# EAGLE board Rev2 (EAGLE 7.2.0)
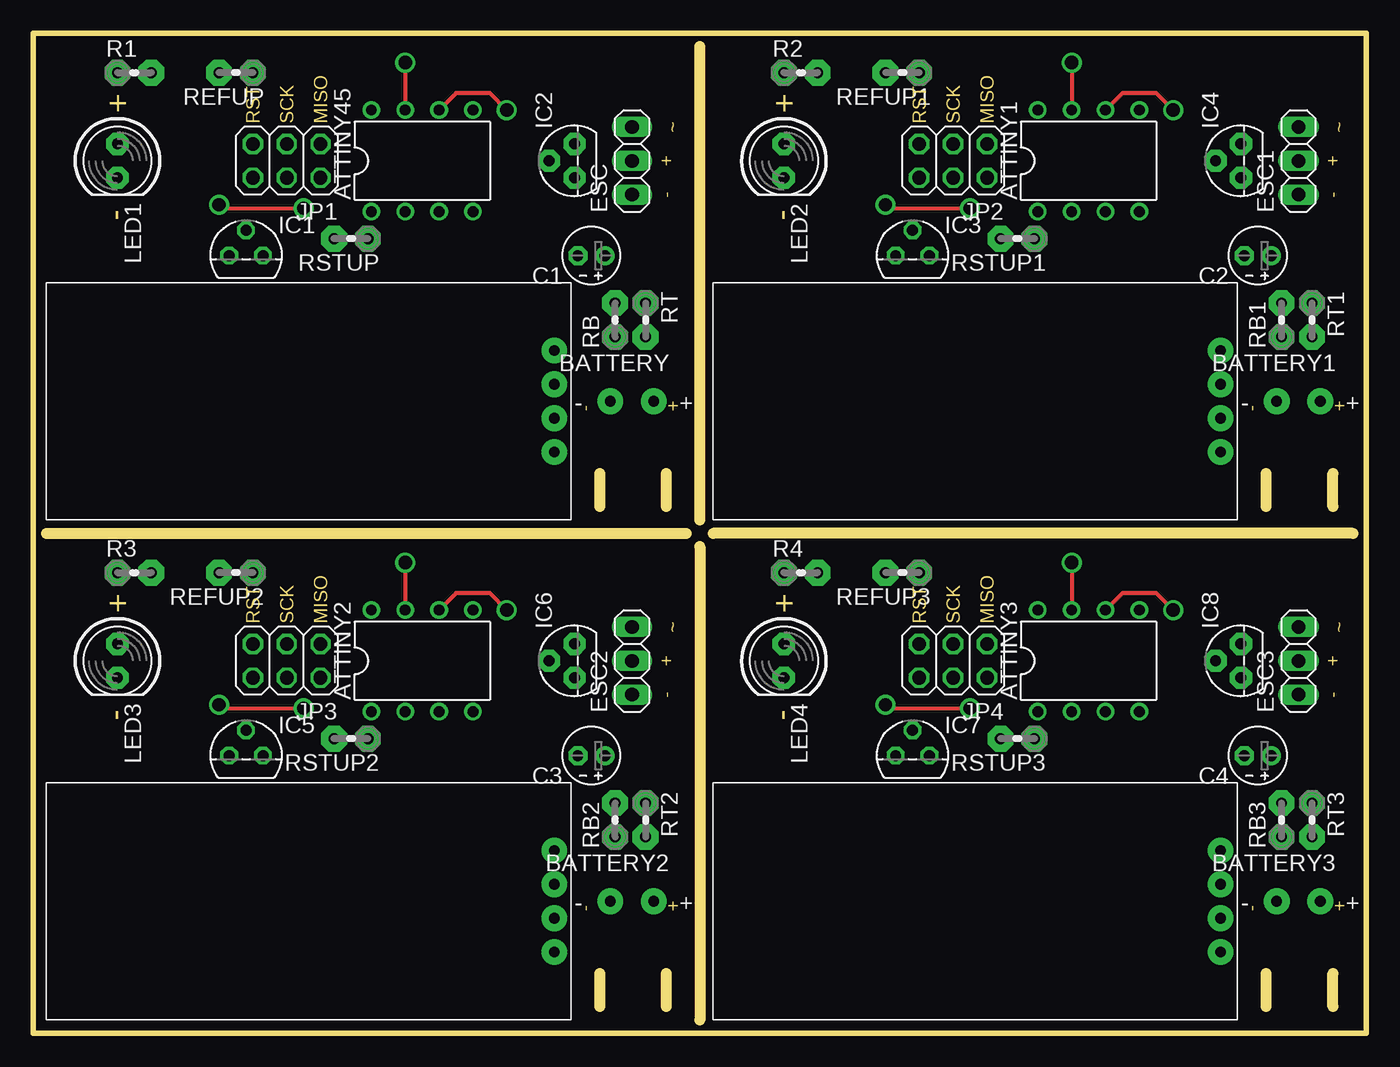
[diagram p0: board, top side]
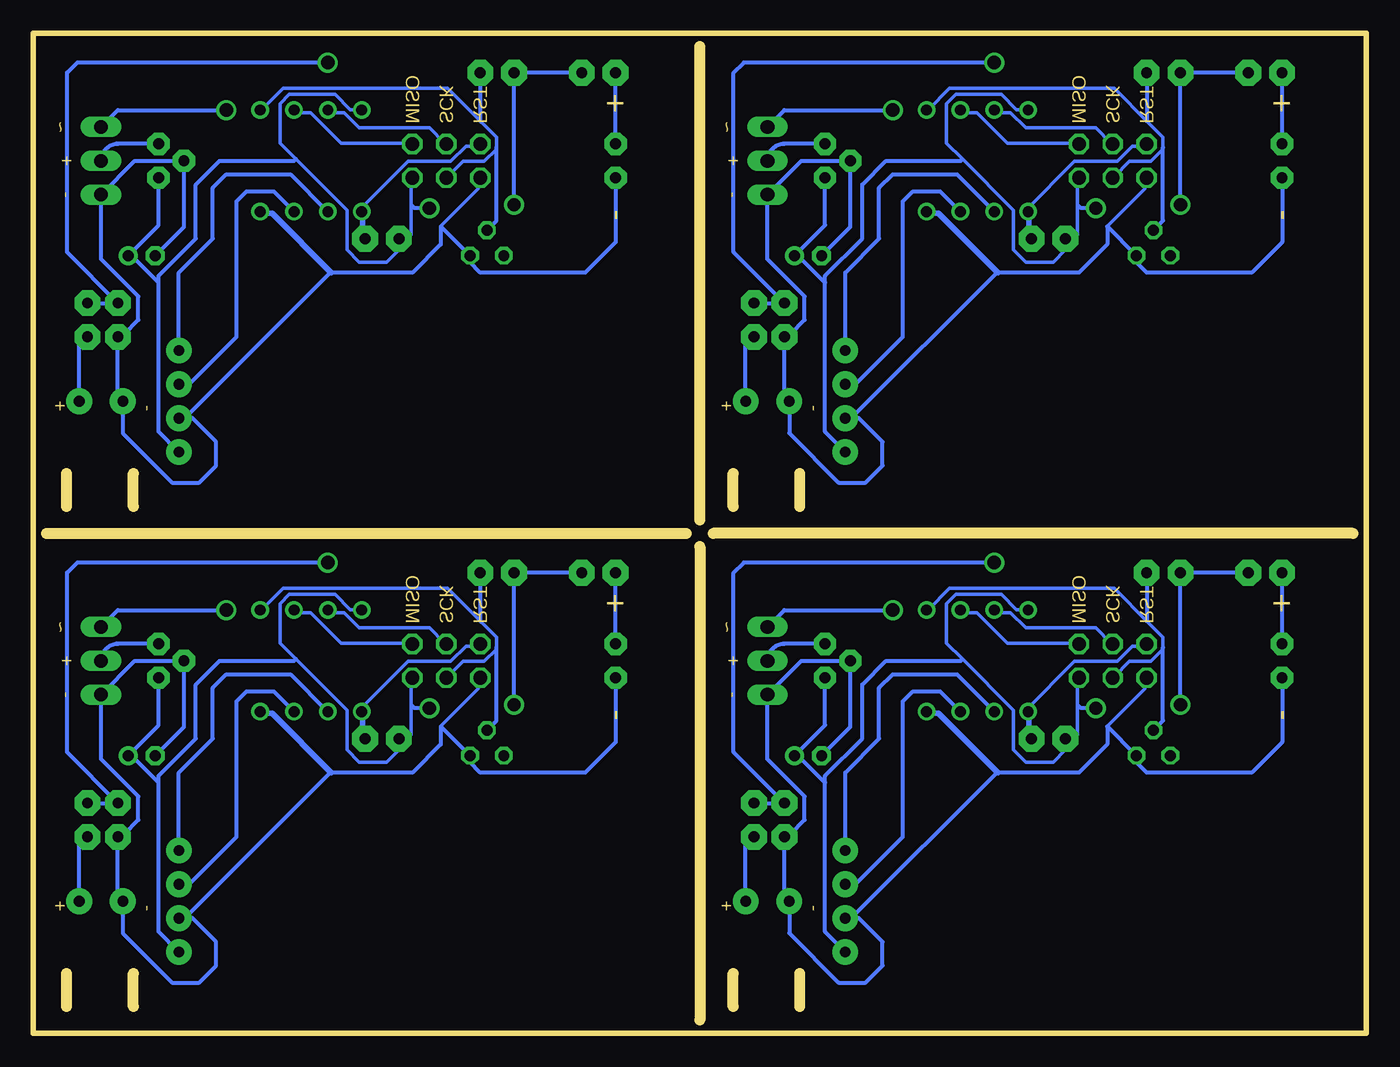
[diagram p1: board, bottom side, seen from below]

Size 100 x 75 mm. Coordinates in mm from the lower left corner, seen from the top.
Outline: 0,75 0,0 100,0 100,75 0,75
Copper layers (1*16): Top 0.035mm / dielectric 1.5mm / Bottom 0.035mm
Design rules "default": minimum track width 10mil, minimum drill 24mil, track to track 8mil, track to pad 8mil, pad to pad 8mil, via to via 8mil, smd to smd 8mil, copper to edge 40mil, drill to drill 8mil, minimum pad ring 10mil, minimum via ring 8mil, stop-mask expansion 4mil, vias tented up to drill 0mil, thermal gap 10mil
Milling: 12 lines

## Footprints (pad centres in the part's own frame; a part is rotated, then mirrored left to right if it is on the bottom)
DIL08 = drill 0.813 pad 1.27: 1 -3.81,-3.81; 2 -1.27,-3.81; 3 1.27,-3.81; 4 3.81,-3.81; 5 3.81,3.81; 6 1.27,3.81; 7 -1.27,3.81; 8 -3.81,3.81
JST-PH-2-THM = drill 0.8 pad 1.93: 1 1.635,0; 2 -1.635,0
E2-4 = drill 0.813 pad 1.422: + -1.016,0 | drill 0.813 pad 1.422 octagon: - 1.016,0
1X03 = drill 1.016 long: 1 -2.54,0; 2 0,0; 3 2.54,0
BT = drill 0.8 pad 1.93: GND -1.27,0; RX 3.81,0; TX 1.27,0; VCC -3.81,0
TO92 = drill 0.813 octagon: 1 -1.27,0; 2 0,1.905; 3 1.27,0
TO92' = drill 0.813 pad 1.676 octagon: 1 -1.27,0; 2 0,1.905; 3 1.27,0
2X03 = drill 1.016 octagon: 1 -2.54,-1.27; 2 -2.54,1.27; 3 0,-1.27; 4 0,1.27; 5 2.54,-1.27; 6 2.54,1.27
LED5MM = drill 0.813 pad 1.676 octagon: A -1.27,0; K 1.27,0
0204V = drill 0.813 pad 1.93 octagon: 1 -1.27,0; 2 1.27,0

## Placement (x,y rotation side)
ATTINY1  ATTINY45DIP8  [DIL08]  79.17,65.44 0 top
ATTINY2  ATTINY45DIP8  [DIL08]  29.17,27.94 0 top
ATTINY3  ATTINY45DIP8  [DIL08]  79.17,27.94 0 top
ATTINY45  ATTINY45DIP8  [DIL08]  29.17,65.44 0 top
BATTERY  [JST-PH-2-THM]  44.92,47.41 180 top
BATTERY1  [JST-PH-2-THM]  94.92,47.41 180 top
BATTERY2  [JST-PH-2-THM]  44.92,9.91 180 top
BATTERY3  [JST-PH-2-THM]  94.92,9.91 180 top
C1  0.1uf  [E2-4]  41.87,58.33 180 top
C2  0.1uf  [E2-4]  91.87,58.33 180 top
C3  0.1uf  [E2-4]  41.87,20.83 180 top
C4  0.1uf  [E2-4]  91.87,20.83 180 top
ESC  [1X03]  44.92,65.44 90 top
ESC1  [1X03]  94.92,65.44 90 top
ESC2  [1X03]  44.92,27.94 90 top
ESC3  [1X03]  94.92,27.94 90 top
HC-01  HC-O6  [BT]  89.08,47.41 90 top
HC-02  HC-O6  [BT]  39.08,9.91 90 top
HC-03  HC-O6  [BT]  89.08,9.91 90 top
HC-06  HC-O6  [BT]  39.08,47.41 90 top
IC1  LM336LP  [TO92]  15.96,58.33 0 top
IC2  78L05Z  [TO92']  40.6,65.44 90 top
IC3  LM336LP  [TO92]  65.96,58.33 0 top
IC4  78L05Z  [TO92']  90.6,65.44 90 top
IC5  LM336LP  [TO92]  15.96,20.83 0 top
IC6  78L05Z  [TO92']  40.6,27.94 90 top
IC7  LM336LP  [TO92]  65.96,20.83 0 top
IC8  78L05Z  [TO92']  90.6,27.94 90 top
JP1  [2X03]  19.01,65.44 180 top
JP2  [2X03]  69.01,65.44 180 top
JP3  [2X03]  19.01,27.94 180 top
JP4  [2X03]  69.01,27.94 180 top
LED1  [LED5MM]  6.31,65.44 270 top
LED2  [LED5MM]  56.31,65.44 270 top
LED3  [LED5MM]  6.31,27.94 270 top
LED4  [LED5MM]  56.31,27.94 270 top
R1  270  [0204V]  7.58,72.04 0 top
R2  270  [0204V]  57.58,72.04 0 top
R3  270  [0204V]  7.58,34.54 0 top
R4  270  [0204V]  57.58,34.54 0 top
RB  20000  [0204V]  43.65,53.5 90 top
RB1  20000  [0204V]  93.65,53.5 90 top
RB2  20000  [0204V]  43.65,16 90 top
RB3  20000  [0204V]  93.65,16 90 top
REFUP  2200  [0204V]  15.2,72.04 180 top
REFUP1  2200  [0204V]  65.2,72.04 180 top
REFUP2  2200  [0204V]  15.2,34.54 180 top
REFUP3  2200  [0204V]  65.2,34.54 180 top
RSTUP  10000  [0204V]  23.84,59.6 180 top
RSTUP1  10000  [0204V]  73.84,59.6 180 top
RSTUP2  10000  [0204V]  23.84,22.1 180 top
RSTUP3  10000  [0204V]  73.84,22.1 180 top
RT  220000  [0204V]  45.94,53.5 270 top
RT1  220000  [0204V]  95.94,53.5 270 top
RT2  220000  [0204V]  45.94,16 270 top
RT3  220000  [0204V]  95.94,16 270 top

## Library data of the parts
ATTINY1-ATTINY3 ATTINY45 HC-01-HC-03 HC-06 IC1 IC3 IC5 IC7 = VLADLIBRARY
BATTERY BATTERY1-BATTERY3 C1-C4 IC2 IC4 IC6 IC8 LED1-LED4 R1-R4 RB RB1-RB3 REFUP REFUP1-REFUP3 RSTUP RSTUP1-RSTUP3 RT RT1-RT3 = adafruit
ESC ESC1-ESC3 JP1-JP4 = pinhead

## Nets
CONTROL: ATTINY45.6 ESC.3 JP1.1
CONTROL1: ATTINY1.6 ESC1.3 JP2.1
CONTROL2: ATTINY2.6 ESC2.3 JP3.1
CONTROL3: ATTINY3.6 ESC3.3 JP4.1
GND: ATTINY45.4 BATTERY.1 C1.- ESC.1 HC-06.GND IC1.3 IC2.2 JP1.6 LED1.K RB.1
GND1: ATTINY1.4 BATTERY1.1 C2.- ESC1.1 HC-01.GND IC3.3 IC4.2 JP2.6 LED2.K RB1.1
GND2: ATTINY2.4 BATTERY2.1 C3.- ESC2.1 HC-02.GND IC5.3 IC6.2 JP3.6 LED3.K RB2.1
GND3: ATTINY3.4 BATTERY3.1 C4.- ESC3.1 HC-03.GND IC7.3 IC8.2 JP4.6 LED4.K RB3.1
N$1: ESC.2 IC2.3
N$2: LED1.A R1.1
N$3: ATTINY45.1 JP1.5 RSTUP.1
N$4: BATTERY.2 RT.2
N$5: ATTINY1.1 JP2.5 RSTUP1.1
N$6: ESC1.2 IC4.3
N$7: BATTERY1.2 RT1.2
N$8: LED2.A R2.1
N$9: ATTINY2.1 JP3.5 RSTUP2.1
N$10: ESC2.2 IC6.3
N$11: BATTERY2.2 RT2.2
N$12: LED3.A R3.1
N$13: ATTINY3.1 JP4.5 RSTUP3.1
N$14: ESC3.2 IC8.3
N$15: BATTERY3.2 RT3.2
N$16: LED4.A R4.1
RX: ATTINY45.3 HC-06.TX
RX1: ATTINY1.3 HC-01.TX
RX2: ATTINY2.3 HC-02.TX
RX3: ATTINY3.3 HC-03.TX
TX: ATTINY45.2 HC-06.RX
TX1: ATTINY1.2 HC-01.RX
TX2: ATTINY2.2 HC-02.RX
TX3: ATTINY3.2 HC-03.RX
VCC: ATTINY45.8 C1.+ HC-06.VCC IC2.1 JP1.2 R1.2 REFUP.2 RSTUP.2
VCC1: ATTINY1.8 C2.+ HC-01.VCC IC4.1 JP2.2 R2.2 REFUP1.2 RSTUP1.2
VCC2: ATTINY2.8 C3.+ HC-02.VCC IC6.1 JP3.2 R3.2 REFUP2.2 RSTUP2.2
VCC3: ATTINY3.8 C4.+ HC-03.VCC IC8.1 JP4.2 R4.2 REFUP3.2 RSTUP3.2
VOLTMETER: ATTINY45.7 JP1.3 RB.2 RT.1
VOLTMETER1: ATTINY1.7 JP2.3 RB1.2 RT1.1
VOLTMETER2: ATTINY2.7 JP3.3 RB2.2 RT2.1
VOLTMETER3: ATTINY3.7 JP4.3 RB3.2 RT3.1
VREF: ATTINY45.5 IC1.2 JP1.4 REFUP.1
VREF1: ATTINY1.5 IC3.2 JP2.4 REFUP1.1
VREF2: ATTINY2.5 IC5.2 JP3.4 REFUP2.1
VREF3: ATTINY3.5 IC7.2 JP4.4 REFUP3.1

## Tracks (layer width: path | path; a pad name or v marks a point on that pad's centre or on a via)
CONTROL  (via drill 1)
  Top 0.305: v35.52,69.25 34.25,70.52 31.71,70.52 ATTINY45.6
  Bottom 0.254: ATTINY45.6 30.34,69.05 29.2,69.05 26.91,66.76 21.65,66.76 JP1.1
  Bottom 0.305: ESC.3 43.65,69.25 v35.52,69.25
CONTROL1  (via drill 1)
  Top 0.305: v85.52,69.25 84.25,70.52 81.71,70.52 ATTINY1.6
  Bottom 0.254: ATTINY1.6 80.34,69.05 79.2,69.05 76.91,66.76 71.65,66.76 JP2.1
  Bottom 0.305: ESC1.3 93.65,69.25 v85.52,69.25
CONTROL2  (via drill 1)
  Top 0.305: v35.52,31.75 34.25,33.02 31.71,33.02 ATTINY2.6
  Bottom 0.254: ATTINY2.6 30.34,31.55 29.2,31.55 26.91,29.26 21.65,29.26 JP3.1
  Bottom 0.305: ESC2.3 43.65,31.75 v35.52,31.75
CONTROL3  (via drill 1)
  Top 0.305: v85.52,31.75 84.25,33.02 81.71,33.02 ATTINY3.6
  Bottom 0.254: ATTINY3.6 80.34,31.55 79.2,31.55 76.91,29.26 71.65,29.26 JP4.1
  Bottom 0.305: ESC3.3 93.65,31.75 v85.52,31.75
GND
  Bottom 0.254: 19.43,60.52 16.62,63.33 16.62,64.02 JP1.6 | 32.85,61.5 ATTINY45.4
  Bottom 0.305: C1.- 38.7,60.49 IC2.2 42.38,65.44 ESC.1 44.92,58.07 42.13,55.28 42.13,53.5 43.14,52.49 43.4,52.49 RB.1 43.65,47.68 BATTERY.1 43.28,45.01 39.59,41.31 37.55,41.31 36.28,42.58 36.28,44.36 38.06,46.14 HC-06.GND 38.65,46.14 27.72,57.06 27.65,57.06 21.55,57.06 19.43,59.18 19.43,60.52 IC1.3 17.23,57.82 16.47,57.06 8.6,57.06 6.31,59.34 LED1.K
  Bottom 0.406: 32.85,61.5 32.09,61.5 27.65,57.06
GND1
  Bottom 0.254: 69.43,60.52 66.62,63.33 66.62,64.02 JP2.6 | 82.86,61.5 ATTINY1.4
  Bottom 0.305: C2.- 88.7,60.49 IC4.2 92.38,65.44 ESC1.1 94.92,58.07 92.13,55.28 92.13,53.5 93.14,52.49 93.4,52.49 RB1.1 93.65,47.68 BATTERY1.1 93.28,45.01 89.59,41.31 87.55,41.31 86.28,42.58 86.28,44.36 88.06,46.14 HC-01.GND 88.65,46.14 77.72,57.06 77.65,57.06 71.55,57.06 69.43,59.18 69.43,60.52 IC3.3 67.23,57.82 66.47,57.06 58.6,57.06 56.31,59.34 LED2.K
  Bottom 0.406: 82.86,61.5 82.09,61.5 77.65,57.06
GND2
  Bottom 0.254: 19.43,23.02 16.62,25.83 16.62,26.52 JP3.6 | 32.85,24 ATTINY2.4
  Bottom 0.305: C3.- 38.7,22.99 IC6.2 42.38,27.94 ESC2.1 44.92,20.57 42.13,17.78 42.13,16 43.14,14.99 43.4,14.99 RB2.1 43.65,10.18 BATTERY2.1 43.28,7.51 39.59,3.81 37.55,3.81 36.28,5.08 36.28,6.86 38.06,8.64 HC-02.GND 38.65,8.64 27.72,19.56 27.65,19.56 21.55,19.56 19.43,21.68 19.43,23.02 IC5.3 17.23,20.32 16.47,19.56 8.6,19.56 6.31,21.84 LED3.K
  Bottom 0.406: 32.85,24 32.09,24 27.65,19.56
GND3
  Bottom 0.254: 69.43,23.02 66.62,25.83 66.62,26.52 JP4.6 | 82.86,24 ATTINY3.4
  Bottom 0.305: C4.- 88.7,22.99 IC8.2 92.38,27.94 ESC3.1 94.92,20.57 92.13,17.78 92.13,16 93.14,14.99 93.4,14.99 RB3.1 93.65,10.18 BATTERY3.1 93.28,7.51 89.59,3.81 87.55,3.81 86.28,5.08 86.28,6.86 88.06,8.64 HC-03.GND 88.65,8.64 77.72,19.56 77.65,19.56 71.55,19.56 69.43,21.68 69.43,23.02 IC7.3 67.23,20.32 66.47,19.56 58.6,19.56 56.31,21.84 LED4.K
  Bottom 0.406: 82.86,24 82.09,24 77.65,19.56
N$1
  Bottom 0.305: IC2.3 43.65,66.71 arc-90 ESC.2
N$2
  Bottom 0.305: LED1.A R1.1
N$3
  Bottom 0.254: 25.31,61.5 ATTINY45.1 25.54,61.73 21.88,65.39 18.68,65.39 17.54,66.53 16.62,66.53 JP1.5
  Bottom 0.406: 25.31,61.5 25.31,59.6 RSTUP.1
N$4
  Bottom 0.305: BATTERY.2 46.55,51.61 RT.2
N$5
  Bottom 0.254: 75.31,61.5 ATTINY1.1 75.54,61.73 71.88,65.39 68.68,65.39 67.54,66.53 66.62,66.53 JP2.5
  Bottom 0.406: 75.31,61.5 75.31,59.6 RSTUP1.1
N$6
  Bottom 0.305: IC4.3 93.65,66.71 arc-90 ESC1.2
N$7
  Bottom 0.305: BATTERY1.2 96.56,51.61 RT1.2
N$8
  Bottom 0.305: LED2.A R2.1
N$9
  Bottom 0.254: 25.31,24 ATTINY2.1 25.54,24.23 21.88,27.89 18.68,27.89 17.54,29.03 16.62,29.03 JP3.5
  Bottom 0.406: 25.31,24 25.31,22.1 RSTUP2.1
N$10
  Bottom 0.305: IC6.3 43.65,29.21 arc-90 ESC2.2
N$11
  Bottom 0.305: BATTERY2.2 46.55,14.11 RT2.2
N$12
  Bottom 0.305: LED3.A R3.1
N$13
  Bottom 0.254: 75.31,24 ATTINY3.1 75.54,24.23 71.88,27.89 68.68,27.89 67.54,29.03 66.62,29.03 JP4.5
  Bottom 0.406: 75.31,24 75.31,22.1 RSTUP3.1
N$14
  Bottom 0.305: IC8.3 93.65,29.21 arc-90 ESC3.2
N$15
  Bottom 0.305: BATTERY3.2 96.56,14.11 RT3.2
N$16
  Bottom 0.305: LED4.A R4.1
RX
  Bottom 0.305: HC-06.TX 38.32,48.68 34.76,52.23 34.76,62.39 34,63.15 31.97,63.15 ATTINY45.3
RX1
  Bottom 0.305: HC-01.TX 88.32,48.68 84.76,52.23 84.76,62.39 84,63.15 81.97,63.15 ATTINY1.3
RX2
  Bottom 0.305: HC-02.TX 38.32,11.18 34.76,14.73 34.76,24.89 34,25.65 31.97,25.65 ATTINY2.3
RX3
  Bottom 0.305: HC-03.TX 88.32,11.18 84.76,14.73 84.76,24.89 84,25.65 81.97,25.65 ATTINY3.3
TX
  Bottom 0.305: HC-06.RX 39.08,57.06 36.54,59.6 36.54,63.41 35.52,64.42 30.7,64.42 ATTINY45.2
TX1
  Bottom 0.305: HC-01.RX 89.08,57.06 86.54,59.6 86.54,63.41 85.52,64.42 80.7,64.42 ATTINY1.2
TX2
  Bottom 0.305: HC-02.RX 39.08,19.56 36.54,22.1 36.54,25.91 35.52,26.92 30.7,26.92 ATTINY2.2
TX3
  Bottom 0.305: HC-03.RX 89.08,19.56 86.54,22.1 86.54,25.91 85.52,26.92 80.7,26.92 ATTINY3.2
VCC  (via drill 1)
  Top 0.305: v13.93,62.14 14.19,61.88 v20.28,61.88
  Bottom 0.254: ATTINY45.8 25.54,69.28 26.23,69.28 27.37,70.42 30.8,70.42 31.48,69.73 31.48,66.76 30.3,65.58 26.45,61.73 26.45,58.76 25.54,57.84 23.48,57.84 22.57,58.76 RSTUP.2 22.57,58.99 21.65,59.9 21.65,62.14 21.65,64.02 JP1.2
  Bottom 0.305: R1.2 REFUP.2 v13.93,62.14 | v20.28,61.88 21.4,61.88 21.65,62.14 | IC2.1 40.6,60.61 C1.+ 42.63,58.33 40.6,56.3 | HC-06.VCC 40.6,45.12 40.6,56.3 | 40.6,56.3 40.6,56.8 37.81,59.6 37.81,63.66 36.03,65.44 30.44,65.44 30.3,65.58
VCC1  (via drill 1)
  Top 0.305: v63.93,62.14 64.19,61.88 v70.28,61.88
  Bottom 0.254: ATTINY1.8 75.54,69.28 76.23,69.28 77.37,70.42 80.8,70.42 81.48,69.73 81.48,66.76 80.3,65.58 76.45,61.73 76.45,58.76 75.54,57.84 73.48,57.84 72.57,58.76 RSTUP1.2 72.57,58.99 71.65,59.9 71.65,62.14 71.65,64.02 JP2.2
  Bottom 0.305: R2.2 REFUP1.2 v63.93,62.14 | v70.28,61.88 71.4,61.88 71.65,62.14 | IC4.1 90.6,60.61 C2.+ 92.63,58.33 90.6,56.3 | HC-01.VCC 90.6,45.12 90.6,56.3 | 90.6,56.3 90.6,56.8 87.81,59.6 87.81,63.66 86.03,65.44 80.44,65.44 80.3,65.58
VCC2  (via drill 1)
  Top 0.305: v13.93,24.64 14.19,24.38 v20.28,24.38
  Bottom 0.254: ATTINY2.8 25.54,31.77 26.23,31.77 27.37,32.92 30.8,32.92 31.48,32.23 31.48,29.26 30.3,28.08 26.45,24.23 26.45,21.26 25.54,20.34 23.48,20.34 22.57,21.26 RSTUP2.2 22.57,21.49 21.65,22.4 21.65,24.64 21.65,26.52 JP3.2
  Bottom 0.305: R3.2 REFUP2.2 v13.93,24.64 | v20.28,24.38 21.4,24.38 21.65,24.64 | IC6.1 40.6,23.11 C3.+ 42.63,20.83 40.6,18.8 | HC-02.VCC 40.6,7.62 40.6,18.8 | 40.6,18.8 40.6,19.3 37.81,22.1 37.81,26.16 36.03,27.94 30.44,27.94 30.3,28.08
VCC3  (via drill 1)
  Top 0.305: v63.93,24.64 64.19,24.38 v70.28,24.38
  Bottom 0.254: ATTINY3.8 75.54,31.77 76.23,31.77 77.37,32.92 80.8,32.92 81.48,32.23 81.48,29.26 80.3,28.08 76.45,24.23 76.45,21.26 75.54,20.34 73.48,20.34 72.57,21.26 RSTUP3.2 72.57,21.49 71.65,22.4 71.65,24.64 71.65,26.52 JP4.2
  Bottom 0.305: R4.2 REFUP3.2 v63.93,24.64 | v70.28,24.38 71.4,24.38 71.65,24.64 | IC8.1 90.6,23.11 C4.+ 92.63,20.83 90.6,18.8 | HC-03.VCC 90.6,7.62 90.6,18.8 | 90.6,18.8 90.6,19.3 87.81,22.1 87.81,26.16 86.03,27.94 80.44,27.94 80.3,28.08
VOLTMETER  (via drill 1 pad 1.27)
  Top 0.305: v27.9,72.81 ATTINY45.7
  Bottom 0.254: ATTINY45.7 27.83,69.05 26.68,69.05 25.54,67.9 20.28,67.9 19.14,66.76 JP1.3
  Bottom 0.305: RT.1 RB.2 47.46,58.58 47.46,72.04 46.7,72.81 v27.9,72.81
VOLTMETER1  (via drill 1 pad 1.27)
  Top 0.305: v77.9,72.81 ATTINY1.7
  Bottom 0.254: ATTINY1.7 77.83,69.05 76.68,69.05 75.54,67.9 70.28,67.9 69.14,66.76 JP2.3
  Bottom 0.305: RT1.1 RB1.2 97.46,58.58 97.46,72.04 96.7,72.81 v77.9,72.81
VOLTMETER2  (via drill 1 pad 1.27)
  Top 0.305: v27.9,35.31 ATTINY2.7
  Bottom 0.254: ATTINY2.7 27.83,31.55 26.68,31.55 25.54,30.4 20.28,30.4 19.14,29.26 JP3.3
  Bottom 0.305: RT2.1 RB2.2 47.46,21.08 47.46,34.54 46.7,35.31 v27.9,35.31
VOLTMETER3  (via drill 1 pad 1.27)
  Top 0.305: v77.9,35.31 ATTINY3.7
  Bottom 0.254: ATTINY3.7 77.83,31.55 76.68,31.55 75.54,30.4 70.28,30.4 69.14,29.26 JP4.3
  Bottom 0.305: RT3.1 RB3.2 97.46,21.08 97.46,34.54 96.7,35.31 v77.9,35.31
VREF
  Bottom 0.254: ATTINY45.5 32.85,69.28 31.25,70.88 18.91,70.88 16.37,68.34 15.25,67.22 15.25,66.46 15.25,66.3 16.17,65.39 17.77,65.39 18.91,64.25 JP1.4
  Bottom 0.305: IC1.2 15.25,60.94 15.25,66.46 | REFUP.1 16.47,68.44 16.37,68.34
VREF1
  Bottom 0.254: ATTINY1.5 82.86,69.28 81.25,70.88 68.91,70.88 66.37,68.34 65.25,67.22 65.25,66.46 65.25,66.3 66.17,65.39 67.77,65.39 68.91,64.25 JP2.4
  Bottom 0.305: IC3.2 65.25,60.94 65.25,66.46 | REFUP1.1 66.47,68.44 66.37,68.34
VREF2
  Bottom 0.254: ATTINY2.5 32.85,31.77 31.25,33.38 18.91,33.38 16.37,30.84 15.25,29.72 15.25,28.96 15.25,28.8 16.17,27.89 17.77,27.89 18.91,26.75 JP3.4
  Bottom 0.305: IC5.2 15.25,23.44 15.25,28.96 | REFUP2.1 16.47,30.94 16.37,30.84
VREF3
  Bottom 0.254: ATTINY3.5 82.86,31.77 81.25,33.38 68.91,33.38 66.37,30.84 65.25,29.72 65.25,28.96 65.25,28.8 66.17,27.89 67.77,27.89 68.91,26.75 JP4.4
  Bottom 0.305: IC7.2 65.25,23.44 65.25,28.96 | REFUP3.1 66.47,30.94 66.37,30.84

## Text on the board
Milling: + | + | RST | SCK | MISO | ~ | RST | SCK | MISO | ~ | + | + | - | - | - | - | - | + | - | + | + | + | RST | SCK | MISO | RST | SCK | MISO | ~ | ~ | + | + | - | - | - | - | - | + | - | +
